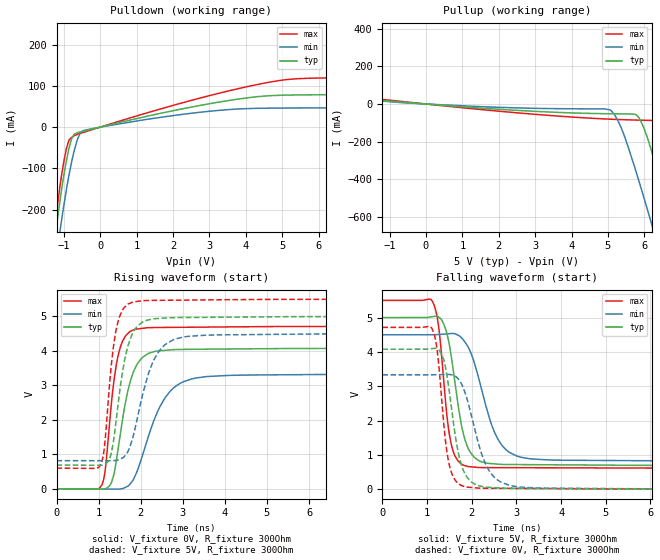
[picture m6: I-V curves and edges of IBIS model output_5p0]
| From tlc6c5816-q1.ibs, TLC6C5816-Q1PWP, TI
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|   output_5p0 Model
[Model]   output_5p0
Model_type   Output
Polarity   Non-Inverting
Vmeas = 2.5
Vref = 0
Cref = 2pF
Rref = 100000
|   typ   min   max
C_comp   2.441pF   2.342pF   2.568pF
|  Where Nom  PVT is Nominal Process, 5.0V,  27C
|   Fast PVT is Strong Process,  5.5V, -40C
|   Slow PVT is Weak Process,   4.5V, 150C
[Voltage Range]   5   4.5   5.5
|Junction Temperature
[Temperature Range]   27   150   -40
[Pullup Reference]   5   4.5   5.5
[Pulldown Reference]   0   0   0
[Power Clamp Reference]   5   4.5   5.5
[GND Clamp Reference]   0   0   0
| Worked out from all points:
|   slope of the pulldown table from 0 to 0.75 V, typ, clamps not added: 47.9 ohm
|   slope of the pullup table from 0 to 0.75 V, typ, clamps not added: 67.3 ohm
|   falling waveform, V_fixture 5V, R_fixture 300Ohm: 20-80 % time 317ps typ, 511ps min, 223ps max; typ from 5 V to 0.687 V
|   rising waveform, V_fixture 0V, R_fixture 300Ohm: 20-80 % time 369ps typ, 634ps min, 256ps max; typ from 0 V to 4.08 V
|   rising waveform, V_fixture 5V, R_fixture 300Ohm: 20-80 % time 323ps typ, 499ps min, 236ps max; typ from 0.687 V to 5 V
|   falling waveform, V_fixture 0V, R_fixture 300Ohm: 20-80 % time 294ps typ, 450ps min, 212ps max; typ from 4.08 V to 0 V
[Pulldown]
|   Voltage   I(typ)   I(min)   I(max)
-5V       -3.039A    -2.915A    -3.137A
-1.25V    -272.7mA   -341.5mA   -239.3mA
-1.1V     -175mA     -248.7mA   -139.5mA
-920mV    -77.51mA   -147.1mA   -49.06mA
-785mV    -28.15mA   -83.93mA   -24.8mA
-620mV    -13.54mA   -28.47mA   -17.34mA
-470mV    -10.01mA   -8.434mA   -12.94mA
4.63V     76.05mA    45.97mA    108.6mA
6.97V     78.8mA     51.97mA    119.8mA
8.2V      80.01mA    83.58mA    120.2mA
9.175V    114.2mA    112mA      134.4mA
10V       257.7mA    241.4mA    269.8mA
[Pullup]
|   Voltage   I(typ)   I(min)   I(max)
-5V       254.7mA    153mA      408mA
-4.07V    99.73mA    91.28mA    183.3mA
-3.53V    82.16mA    76.53mA    93.47mA
5.05V     -51.9mA    -30.76mA   -80.81mA
5.365V    -52.56mA   -127.1mA   -83.26mA
5.845V    -71.02mA   -406.3mA   -85.94mA
6.25V     -283.4mA   -672.3mA   -88.19mA
6.52V     -470mA     -853.8mA   -127mA
6.85V     -706.9mA   -1.078A    -327.6mA
7.225V    -980.6mA   -1.335A    -605.3mA
7.405V    -1.113A    -1.459A    -742.1mA
10V       -3.042A    -3.265A    -2.755A
[Ramp]
R_load = 300
|   typ   min   max
dV/dt_r   2.44718/3.68717e-10   1.99905/6.32905e-10   2.82805/2.56422e-10
dV/dt_f   2.58792/3.1727e-10   2.2112/5.11057e-10   2.94116/2.23232e-10
[Falling Waveform]
V_fixture = 5V
V_fixture_min = 4.5V
V_fixture_max = 5.5V
R_fixture = 300Ohm
C_fixture = 0F
|   Time   V(typ)   V(min)   V(max)
0s        5V         4.5V       5.5V
1.118ns   5.025V     4.5V       5.481V
1.26ns    5.018V     4.507V     4.731V
1.375ns   4.808V     4.518V     3.153V
1.578ns   3.549V     4.538V     1.132V
1.819ns   1.585V     4.342V     697.9mV
2.147ns   843.7mV    3.28V      631.8mV
2.704ns   721mV      1.235V     626.6mV
3.88ns    709.5mV    846.7mV    622.2mV
100ns     686.8mV    814.7mV    598.1mV
[Rising Waveform]
V_fixture = 0V
V_fixture_min = 0V
V_fixture_max = 0V
R_fixture = 300Ohm
C_fixture = 0F
|   Time   V(typ)   V(min)   V(max)
0s        -119.7nV   -399.6nV   -12.68nV
1.075ns   -11.46mV   -8.472mV   107.7mV
1.159ns   1.195mV    -9.133mV   570mV
1.311ns   202.1mV    -10.33mV   2.557V
1.5ns     1.452V     -8.828mV   4.037V
1.787ns   3.25V      200.2mV    4.585V
2.147ns   3.896V     1.374V     4.668V
2.848ns   4.036V     2.987V     4.68V
4.307ns   4.054V     3.292V     4.695V
100ns     4.079V     3.332V     4.713V
[Rising Waveform]
V_fixture = 5V
V_fixture_min = 4.5V
V_fixture_max = 5.5V
R_fixture = 300Ohm
C_fixture = 0F
|   Time   V(typ)   V(min)   V(max)
0s        686.8mV    814.7mV    598.1mV
1.041ns   680.7mV    814.6mV    675.8mV
1.14ns    697.9mV    814.3mV    1.225V
1.293ns   995.4mV    813.9mV    3.471V
1.462ns   2.434V     831.8mV    4.845V
1.7ns     4.152V     1.09V      5.356V
2.062ns   4.846V     2.811V     5.454V
2.579ns   4.951V     4.178V     5.465V
3.88ns    4.973V     4.462V     5.479V
100ns     5V         4.5V       5.5V
[Falling Waveform]
|Gnd
V_fixture = 0V
V_fixture_min = 0V
V_fixture_max = 0V
R_fixture = 300Ohm
C_fixture = 0F
|   Time   V(typ)   V(min)   V(max)
0s        4.079V     3.332V     4.713V
1.105ns   4.095V     3.332V     4.696V
1.224ns   4.097V     3.335V     4.082V
1.361ns   3.82V      3.341V     2.109V
1.524ns   2.605V     3.338V     580.1mV
1.787ns   638.4mV    3.026V     98.13mV
2.147ns   103.7mV    1.351V     31.56mV
2.64ns    31.79mV    214.1mV    24.06mV
3.88ns    19.34mV    24.45mV    15.31mV
100ns     -120.3nV   -426.9nV   -12.68nV
